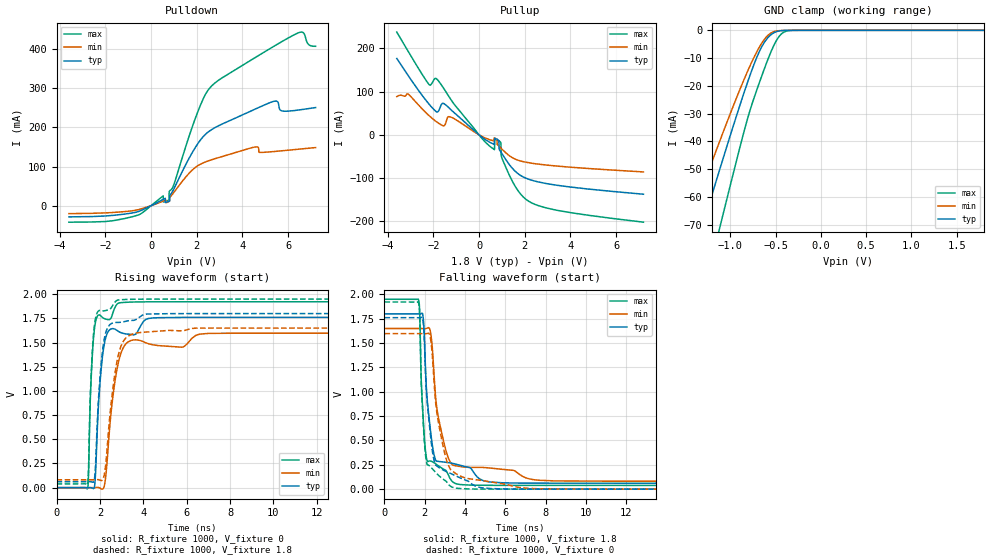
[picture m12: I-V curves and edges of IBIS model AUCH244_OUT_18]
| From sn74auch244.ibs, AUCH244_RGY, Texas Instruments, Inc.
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[Model]   AUCH244_OUT_18
Model_type  3-state
Enable   Active-Low
Vref =   0
Rref =   1000
Cref =   30p
Vmeas =   0.9
| variable   typ   min   max
C_comp   5.69pF   5.12pF   5.95pF
| C_pullup   6.46pF   0.71pF   12.07pF
| C_pulldown   6.31pF   1.58pF   14.05pF
| C_tri-state   5.69pF   5.12pF   5.95pF
[Temperature Range]   40   100   -40
| Ambient temperature   25   85   -40
[Voltage range]   1.8   1.65   1.95
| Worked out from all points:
|   slope of the pulldown table from 0 to 0.27 V, typ, clamps not added: 34.2 ohm
|   slope of the pullup table from 0 to 0.27 V, typ, clamps not added: 24.6 ohm
|   GND clamp passes 1 mA (typ) near -0.53 V on its own axis
|   rising waveform, R_fixture 1000, V_fixture 0: 20-80 % time 313ps typ, 487ps min, 202ps max; typ from 0 V to 1.76 V
|   falling waveform, R_fixture 1000, V_fixture 1.8: 20-80 % time 407ps typ, 640ps min, 246ps max; typ from 1.8 V to 0.061 V
|   rising waveform, R_fixture 1000, V_fixture 1.8: 20-80 % time 311ps typ, 486ps min, 200ps max; typ from 0.061 V to 1.8 V
|   falling waveform, R_fixture 1000, V_fixture 0: 20-80 % time 409ps typ, 643ps min, 244ps max; typ from 1.76 V to 0 V
[GND Clamp]
| AUCH244_OUT_18
|   Voltage   I(typ)   I(min)   I(max)
-3.6V     -322.8mA   -271.3mA   -392.8mA
-1.48V    -89.12mA   -71.98mA   -118.6mA
-1.435V   -84.22mA   -67.92mA   -112.7mA
-1.3V     -69.58mA   -55.84mA   -94.96mA
-1.15V    -53.48mA   -42.67mA   -75.27mA
-1.1V     -48.18mA   -38.36mA   -68.71mA
-830mV    -20.57mA   -16.22mA   -34.06mA
-690mV    -8.335mA   -6.603mA   -19.75mA
-565mV    -1.951mA   -1.255mA   -8.764mA
-490mV    -463.9uA   -245.8uA   -3.576mA
-425mV    -91.38uA   -54.14uA   -985.3uA
1.8V      674.8pA    50.14nA    728.7pA
[Pulldown]
| AUCH244_OUT_18
|   Voltage   I(typ)   I(min)   I(max)
-3.6V     -28.49mA   -20.22mA   -42.08mA
-1.15V    -21.28mA   -15.02mA   -32.6mA
530mV     16.28mA    11.83mA    25.26mA
780mV     11.06mA    10.81mA    14.1mA
800mV     11.7mA     11.72mA    36.72mA
1.955V    150.3mA    98.42mA    225.9mA
2.625V    193.2mA    116.8mA    304mA
4.56V     246.5mA    149.9mA    378.1mA
5.38V     266.4mA    138.3mA    406.9mA
5.71V     242.1mA    140mA      418.2mA
6.445V    244.1mA    144.1mA    441.1mA
7.2V      250.4mA    148.3mA    406.7mA
[Pullup]
| AUCH244_OUT_18
|   Voltage   I(typ)   I(min)   I(max)
-3.6V     176.5mA    88.25mA    237.5mA
-2.185V   70.84mA    44.34mA    116.3mA
-1.835V   52.55mA    29.22mA    128.3mA
-1.53V    71.89mA    20.76mA    106.1mA
-1.26V    59.61mA    41.57mA    83.77mA
480mV     -17.54mA   -11.58mA   -26.82mA
845mV     -12.07mA   -24.67mA   -13.29mA
940mV     -38.23mA   -29.59mA   -16.84mA
980mV     -41.44mA   -31.73mA   -49.64mA
1.255V    -63.59mA   -45.3mA    -84.99mA
2.06V     -100.4mA   -63.37mA   -149.4mA
7.2V      -137.4mA   -85.82mA   -202mA
[Ramp]
| AUCH244_OUT_18
| variable   typ   min   max
dV/dt_r   1.06/3.14E-10   0.97/4.92E-10   1.16/2.02E-10
dV/dt_f   1.05/4.10E-10   0.95/6.43E-10   1.15/2.47E-10
R_load = 1000
[Rising Waveform]
| AUCH244_OUT_18
R_fixture =   1000
C_fixture =   0
L_fixture =   0
V_fixture =   0
V_fixture_min = 0
V_fixture_max = 0
|   Time   V(typ)   V(min)   V(max)
0s        10.65nV    37.28nV    1.248nV
1.43ns    69uV       -8.908uV   -5.32mV
1.475ns   329.2uV    -11.78uV   143mV
1.57ns    151.2uV    -15.01uV   990.8mV
1.72ns    -6.286mV   227.2uV    1.583V
1.975ns   995.7mV    -1.786mV   1.786V
2.17ns    1.441V     -3.239mV   1.752V
2.905ns   1.609V     1.343V     1.911V
7.01ns    1.761V     1.595V     1.922V
34.99ns   1.761V     1.597V     1.922V
[Falling Waveform]
| AUCH244_OUT_18
R_fixture =   1000
C_fixture =   0
L_fixture =   0
V_fixture =   1.8
V_fixture_min = 1.65
V_fixture_max = 1.95
|   Time   V(typ)   V(min)   V(max)
0s        1.8V       1.65V      1.95V
1.68ns    1.8V       1.65V      1.952V
1.74ns    1.799V     1.65V      1.864V
1.925ns   1.76V      1.649V     726.9mV
2.1ns     984.2mV    1.652V     305.2mV
2.32ns    544.7mV    1.568V     287.1mV
2.535ns   302.7mV    962.9mV    261.1mV
3.09ns    274.8mV    371mV      181.3mV
3.595ns   254.6mV    238.2mV    53.72mV
34.99ns   61.09mV    81.02mV    38.7mV
[Rising Waveform]
| AUCH244_OUT_18
R_fixture =   1000
C_fixture =   0
L_fixture =   0
V_fixture =   1.8
V_fixture_min = 1.65
V_fixture_max = 1.95
|   Time   V(typ)   V(min)   V(max)
0s        61.05mV    81.01mV    38.68mV
1.425ns   61.11mV    81mV       32.41mV
1.47ns    61.33mV    81mV       162.4mV
1.575ns   61.22mV    81mV       1.054V
1.725ns   66.97mV    81.26mV    1.635V
1.96ns    1.002V     80.91mV    1.831V
2.17ns    1.497V     105mV      1.828V
2.845ns   1.708V     1.367V     1.941V
6.43ns    1.8V       1.65V      1.95V
34.99ns   1.8V       1.65V      1.95V
[Falling Waveform]
| AUCH244_OUT_18
R_fixture =   1000
C_fixture =   0
L_fixture =   0
V_fixture =   0
V_fixture_min = 0
V_fixture_max = 0
|   Time   V(typ)   V(min)   V(max)
0s        1.761V     1.597V     1.922V
1.68ns    1.76V      1.597V     1.924V
1.74ns    1.76V      1.597V     1.833V
1.92ns    1.724V     1.596V     714mV
2.09ns    982.3mV    1.597V     277.7mV
2.305ns   518.2mV    1.52V      226.2mV
2.505ns   267.4mV    982.9mV    180.6mV
2.985ns   189.1mV    375.2mV    92.45mV
3.435ns   147.3mV    175.8mV    15.96mV
34.99ns   36.21uV    2.964uV    15.49uV
